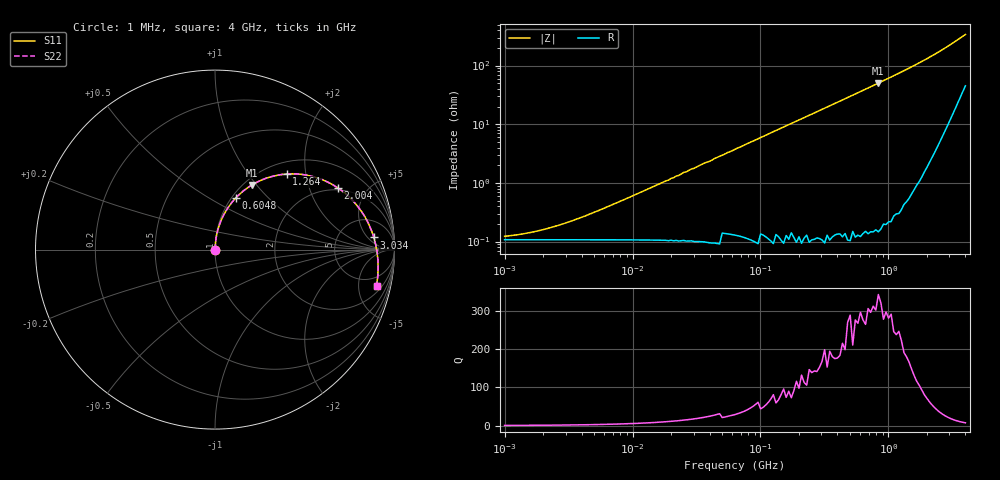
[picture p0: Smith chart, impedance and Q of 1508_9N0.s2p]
# MHz S MA R 50
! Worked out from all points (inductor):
!   181 points, 1 MHz to 4 GHz, reference 50 ohm
!   read as one part in series: L = 9.39 nH near 5.501 MHz
!   highest Q = 321 at 835 MHz (marker M1), where L = 9.57 nH
!   S11 on the Smith chart (normalised r, x): 1 MHz: 1.00, +0.00; 604.8 MHz: 1.05, +0.67; 1.264 GHz: 1.23, +1.56; 2.004 GHz: 1.91, +3.18; 3.034 GHz: 12, +8; 4 GHz: 2.99, -7.99
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1  0.001268 25.0  0.999 -0.0  0.999 -0.0  0.001268 25.0
2.09  0.001606 44.3  0.999 -0.1  0.999 -0.1  0.001607 44.3
4.172  0.002518 62.7  0.999 -0.2  0.999 -0.2  0.002519 62.7
16.623  0.009002 82.1  0.999 -0.6  0.999 -0.6  0.009006 82.1
21.916  0.012 83.6  0.999 -0.8  0.999 -0.8  0.012 83.6
22.95  0.012 83.8  0.999 -0.8  0.999 -0.8  0.012 83.8
25.165  0.014 84.2  0.999 -0.9  0.999 -0.9  0.014 84.2
26.352  0.014 84.4  0.999 -1.0  0.999 -1.0  0.014 84.4
63.246  0.034 85.7  0.998 -2.3  0.998 -2.3  0.034 85.7
138.428  0.074 84.0  0.996 -5.1  0.996 -5.1  0.074 84.0
263.867  0.141 79.9  0.989 -9.7  0.989 -9.7  0.141 79.9
418.311  0.22 74.5  0.974 -15.2  0.974 -15.2  0.22 74.5
604.771  0.312 67.9  0.949 -21.8  0.949 -21.8  0.312 67.9
834.97  0.416 60.1  0.908 -29.7  0.908 -29.7  0.417 60.1
1003.961  0.486 54.6  0.872 -35.1  0.872 -35.1  0.486 54.6
1264.078  0.58 46.6  0.812 -43.1  0.812 -43.1  0.58 46.6
1591.59  0.676 37.2  0.731 -52.3  0.731 -52.3  0.676 37.2
2003.957  0.767 26.5  0.63 -62.6  0.63 -62.6  0.767 26.5
2409.54  0.829 17.1  0.537 -71.3  0.537 -71.3  0.83 17.1
3033.831  0.888 4.4  0.413 -82.4  0.413 -82.4  0.888 4.4
3483.579  0.91 -3.8  0.341 -88.7  0.341 -88.7  0.91 -3.8
4000  0.922 -12.6  0.275 -94.3  0.275 -94.3  0.923 -12.6
